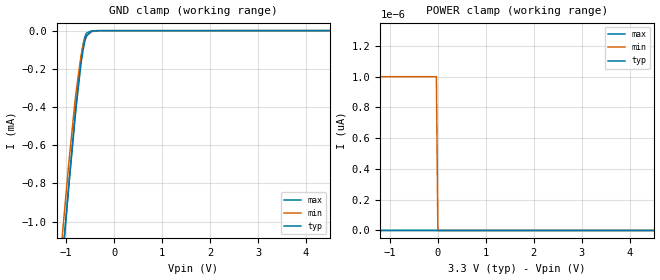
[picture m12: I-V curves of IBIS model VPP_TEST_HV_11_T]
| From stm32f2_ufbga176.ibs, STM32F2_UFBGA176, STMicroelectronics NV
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| *** New cell (Generated with 5.14beta1 (Sep 20 2010 13:23:23))
[Model]   VPP_TEST_HV_11_T
Model_type Input
Polarity   Non-Inverting
Enable   Active-Low
| CAP_THRESHOLD on pad VPPHV is "CMOS" :
| Rising=10.0% of vddio   Falling=90.0% of vddio
| C_comp min and max val. don't necessarily correlate with the min and max pvt
| but are the smallest and greatest pad capacitance found.
| var   typ   min   max
C_comp   1.28660pF  1.28345pF  1.28875pF
Vinl = 810.0mV | Dummy value overriden by next lines
Vinh = 2.52V | Dummy value overriden by next lines
[Model Spec]
| TIME_THRESHOLD on pin ZIV33 is "CORE" :
| Rising=40.0% of vddio   Falling=60.0% of vddio
Vinl 746.50000mV 616.50000mV 806.50000mV
Vinh 911.50000mV 803.50000mV 950.50000mV
| variable   typ   min   max
[Temperature Range] 25.0 125.0 -40.0
| variable   typ   min   max
[Voltage Range] 3.3V 2.7V 3.6V
| variable   typ   min   max
[POWER Clamp Reference] 3.3V 2.7V 3.6V
| variable   typ   min   max
[GND Clamp Reference] 0V 0V 0V
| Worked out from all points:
|   GND clamp passes 1 mA (typ) near -1.01 V on its own axis
[POWER Clamp]
-3.3V     8.2nA      26pA       28.98nA
-3.27V    7.66nA     2pA        27.33nA
-3.26V    7.49nA     1pA        26.8nA
-2.5V     10pA       1pA        2.99nA
-2.47V    0A         1pA        2.57nA
-2.22V    0A         1pA        40pA
-2.21V    0A         1pA        0A
-30mV     0A         1pA        0A
0V        0A         0A         0A
6.6V      0A         0A         0A
[GND Clamp]
-3.3V     -8.344mA   -8.255mA   -8.245mA
-1.18V    -1.518mA   -1.372mA   -1.509mA
-1.06V    -1.156mA   -1.018mA   -1.147mA
-940mV    -805.4uA   -683.6uA   -793.9uA
-820mV    -477.2uA   -383.4uA   -459.2uA
-790mV    -400.8uA   -316.9uA   -380.6uA
-700mV    -196.2uA   -149.7uA   -168.8uA
-650mV    -107.7uA   -84.49uA   -79.68uA
-600mV    -47.2uA    -42.16uA   -26.45uA
-570mV    -25.73uA   -26.52uA   -11.89uA
-470mV    -2.603uA   -5.115uA   -823.2nA
6.6V      182.5nA    50.74nA    482.8nA
